[IBIS Ver]  4.0
[File Name]  lpc2478fbd.ibs
[File Rev]  1.0
[Date]  Mon Dec 18 10:34:29 2006
[Source]  Package model from Ansoft Q3D Extractor 7.1.1
[Notes]   IO models Rev 0.20 IBIS Model Design Automation Generation
[Copyright]  NXP Semiconductors 2006,2007. All rights reserved.
|   lpc2478FBD (208 LOFP package) IBIS Model
[Disclaimer]
| NXP Semiconductors warrants and represents that the IBIS models
| identified herein are owned by NXP Semiconductors (NXP).  The
| models provided are not warranted as fully representing all of the
| operating characteristics and specifications of the semiconductor
| products to which the models relate.  Moreover, unless there is a
| signed, written agreement to the contrary, these models are furnished
| on an "as is" basis without support or warranty of any kind, either
| expressed or implied, regarding the use thereof, and NXP
| specifically disclaims all implied warranties of merchantability and
| fitness of the models for any purpose.
| NXP does not assume any liability arising out of the application
| or use of these IBIS models including infringement of patents and
| copyrights, nor does NXP convey any license under its patents and
| copyrights or the rights of others.
| NXP provides IBIS models as a service to our customers.  You and
| your company shall not distribute, convey, sell, or give these models
| to anyone else without receiving prior written permission from
| NXP.
[Define Package Model]  LQFP208
[Manufacturer]  NXP Semiconductors
[OEM]  NXP
[Description]  LQFP208
|Sim freq: 100 MHz
|Date: 121806
[Number Of Pins]  208
[Pin Numbers]
1   | pin1 = lead1
2   | pin2 = lead2
3   | pin3 = lead3
4   | pin4 = lead4
5   | pin5 = lead5
6   | pin6 = lead6
7   | pin7 = lead7
8   | pin8 = lead8
9   | pin9 = lead9
10   | pin10 = lead10
11   | pin11 = lead11
12   | pin12 = lead12
13   | pin13 = lead13
14   | pin14 = lead14
15   | pin15 = lead15
16   | pin16 = lead16
17   | pin17 = lead17
18   | pin18 = lead18
19   | pin19 = lead19
20   | pin20 = lead20
21   | pin21 = lead21
22   | pin22 = lead22
23   | pin23 = lead23
24   | pin24 = lead24
25   | pin25 = lead25
26   | pin26 = lead26
27   | pin27 = lead27
28   | pin28 = lead28
29   | pin29 = lead29
30   | pin30 = lead30
31   | pin31 = lead31
32   | pin32 = lead32
33   | pin33 = lead33
34   | pin34 = lead34
35   | pin35 = lead35
36   | pin36 = lead36
37   | pin37 = lead37
38   | pin38 = lead38
39   | pin39 = lead39
40   | pin40 = lead40
41   | pin41 = lead41
42   | pin42 = lead42
43   | pin43 = lead43
44   | pin44 = lead44
45   | pin45 = lead45
46   | pin46 = lead46
47   | pin47 = lead47
48   | pin48 = lead48
49   | pin49 = lead49
50   | pin50 = lead50
51   | pin51 = lead51
52   | pin52 = lead52
53   | pin53 = lead53
54   | pin54 = lead54
55   | pin55 = lead55
56   | pin56 = lead56
57   | pin57 = lead57
58   | pin58 = lead58
59   | pin59 = lead59
60   | pin60 = lead60
61   | pin61 = lead61
62   | pin62 = lead62
63   | pin63 = lead63
64   | pin64 = lead64
65   | pin65 = lead65
66   | pin66 = lead66
67   | pin67 = lead67
68   | pin68 = lead68
69   | pin69 = lead69
70   | pin70 = lead70
71   | pin71 = lead71
72   | pin72 = lead72
73   | pin73 = lead73
74   | pin74 = lead74
75   | pin75 = lead75
76   | pin76 = lead76
77   | pin77 = lead77
78   | pin78 = lead78
79   | pin79 = lead79
80   | pin80 = lead80
81   | pin81 = lead81
82   | pin82 = lead82
83   | pin83 = lead83
84   | pin84 = lead84
85   | pin85 = lead85
86   | pin86 = lead86
87   | pin87 = lead87
88   | pin88 = lead88
89   | pin89 = lead89
90   | pin90 = lead90
91   | pin91 = lead91
92   | pin92 = lead92
93   | pin93 = lead93
94   | pin94 = lead94
95   | pin95 = lead95
96   | pin96 = lead96
97   | pin97 = lead97
98   | pin98 = lead98
99   | pin99 = lead99
100   | pin100 = lead100
101   | pin101 = lead101
102   | pin102 = lead102
103   | pin103 = lead103
104   | pin104 = lead104
105   | pin105 = lead105
106   | pin106 = lead106
107   | pin107 = lead107
108   | pin108 = lead108
109   | pin109 = lead109
110   | pin110 = lead110
111   | pin111 = lead111
112   | pin112 = lead112
113   | pin113 = lead113
114   | pin114 = lead114
115   | pin115 = lead115
116   | pin116 = lead116
117   | pin117 = lead117
118   | pin118 = lead118
119   | pin119 = lead119
120   | pin120 = lead120
121   | pin121 = lead121
122   | pin122 = lead122
123   | pin123 = lead123
124   | pin124 = lead124
125   | pin125 = lead125
126   | pin126 = lead126
127   | pin127 = lead127
128   | pin128 = lead128
129   | pin129 = lead129
130   | pin130 = lead130
131   | pin131 = lead131
132   | pin132 = lead132
133   | pin133 = lead133
134   | pin134 = lead134
135   | pin135 = lead135
136   | pin136 = lead136
137   | pin137 = lead137
138   | pin138 = lead138
139   | pin139 = lead139
140   | pin140 = lead140
141   | pin141 = lead141
142   | pin142 = lead142
143   | pin143 = lead143
144   | pin144 = lead144
145   | pin145 = lead145
146   | pin146 = lead146
147   | pin147 = lead147
148   | pin148 = lead148
149   | pin149 = lead149
150   | pin150 = lead150
151   | pin151 = lead151
152   | pin152 = lead152
153   | pin153 = lead153
154   | pin154 = lead154
155   | pin155 = lead155
156   | pin156 = lead156
157   | pin157 = lead157
158   | pin158 = lead158
159   | pin159 = lead159
160   | pin160 = lead160
161   | pin161 = lead161
162   | pin162 = lead162
163   | pin163 = lead163
164   | pin164 = lead164
165   | pin165 = lead165
166   | pin166 = lead166
167   | pin167 = lead167
168   | pin168 = lead168
169   | pin169 = lead169
170   | pin170 = lead170
171   | pin171 = lead171
172   | pin172 = lead172
173   | pin173 = lead173
174   | pin174 = lead174
175   | pin175 = lead175
176   | pin176 = lead176
177   | pin177 = lead177
178   | pin178 = lead178
179   | pin179 = lead179
180   | pin180 = lead180
181   | pin181 = lead181
182   | pin182 = lead182
183   | pin183 = lead183
184   | pin184 = lead184
185   | pin185 = lead185
186   | pin186 = lead186
187   | pin187 = lead187
188   | pin188 = lead188
189   | pin189 = lead189
190   | pin190 = lead190
191   | pin191 = lead191
192   | pin192 = lead192
193   | pin193 = lead193
194   | pin194 = lead194
195   | pin195 = lead195
196   | pin196 = lead196
197   | pin197 = lead197
198   | pin198 = lead198
199   | pin199 = lead199
200   | pin200 = lead200
201   | pin201 = lead201
202   | pin202 = lead202
203   | pin203 = lead203
204   | pin204 = lead204
205   | pin205 = lead205
206   | pin206 = lead206
207   | pin207 = lead207
208   | pin208 = lead208
[Model Data]
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[End Model Data]
[End Package Model]
|| [End]
[Component]   lpc2478FBD
[Manufacturer]  NXP
[Package]
|   typ   min   max
R_pkg   0   0   0  |Values included in package model
L_pkg   0   0   0  |Values included in package model
C_pkg   0   0   0  |Values included in package model
[Package Model]  LQFP208
| (Pin and IO model definitions)
| IMPORTANT NOTES:
| The lpc2478 GPIO pins, excluding the I2C and USB, have programmable input
| configurations. For this reason, three models are supplied for those basic
| padcells. Each model is identified by a unique suffix code at the end of
| the modelname:
| _p=plain input, _pd=pulldown enabled, _pu=pullup enabled
| The model_name for each of the GPIO pins in the [Pin] table below reflects
| the default state of that pin on power up (input with pullup enabled).
| The user may modify the model_name for a specific P#.# pin if that pin's
| input configuration is programmed differently from the default in the
| actual application. However, the model_names for all other pins are
| non-configurable and should not be altered.
| All GPIO padcells have 5ns slew rate control when operated as outputs,
| unless otherwise noted.
[Pin]   signal_name   model_name   | comments
1   P3.12   bpts5ptpht5v_pu   |
2   TDO   bpts5ptpht5v_p   | 3-state output only
3   P3.3   bpts5ptpht5v_pu   |
4   TDI   bpts5ptpht5v_pu   | In only
5   P3.28   bpts5ptpht5v_pu   |
6   TMS   bpts5ptpht5v_pu   | In only
7   P3.13   bpts5ptpht5v_pu   |
8   TRST_N   bpts5ptpht5v_pu   | In only
9   DBGEN   bpts5ptpht5v_pu   | In only
10   TCK   bpts5ptpht5v_p   | In only
11   P3.29   bpts5ptpht5v_pu   |
12   P0.26   bpats5thpept5v_pu |
13   P3.4   bpts5ptpht5v_pu   |
14   P0.25   bpats5thpept5v_pu |
15   Vdd   POWER
16   P0.24   bpats5thpept5v_pu |
17   P3.5   bpts5ptpht5v_pu   |
18   P0.23   bpats5thpept5v_pu |
19   P3.30   bpts5ptpht5v_pu   |
20   VddA   POWER
21   P3.14   bpts5ptpht5v_pu   |
22   VssA   GND
23   P3.6   bpts5ptpht5v_pu   |
24   VrefA   POWER
25   P3.31   bpts5ptpht5v_pu   |
26   Vdd   POWER   |
27   P3.7   bpts5ptpht5v_pu   |
28   P3.15   bpts5ptpht5v_pu   |
29   RSTOUTN   bpts5ptpht5v_pu   | Output only
30   Vddcore   NC   |
31   P2.30   bpts5ptpht5v_pu   |
32   Vss   GND
33   Vss   GND
34   RTCX1   NC
35   NRESET   bpts5ptpht5v_pu   | In only
36   RTCX2   NC
37   ALARM   bptpcph1v8   | Output only, 1.8V, no slew
38   VBAT   POWER
39   P2.31   bpts5ptpht5v_pu   |
40   P1.31   bpats5thpept5v_pu |
41   P0.12   bpats5thpept5v_pu |
42   P1.30   bpats5thpept5v_pu |
43   P2.29   bpts5ptpht5v_pu   |
44   X1   NC
45   P0.13   bpats5thpept5v_pu |
46   X2   NC
47   P2.27   bpts5ptpht5v_pu   |
48   P0.28   iic3m4sdat5v_400k | I2C padcell
49   P2.28   bpts5ptpht5v_pu   |
50   P0.27   iic3m4sdat5v_400k | I2C padcell
51   P0.31   usb11f1_iop_hs   | USB padcell
52   DMB   usb11f1_iom_hs   | USB padcell
53   P2.24   bpts5ptpht5v_pu   |
54   P2.25   bpts5ptpht5v_pu   |
55   P3.26   bpts5ptpht5v_pu   |
56   P3.25   bpts5ptpht5v_pu   |
57   P2.26   bpts5ptpht5v_pu   |
58   P3.24   bpts5ptpht5v_pu   |
59   P2.18   bpts5ptpht5v_pu   |
60   Vdd   POWER
61   P0.29   usb11f1_iop_hs   | USB padcell
62   P0.30   usb11f1_iom_hs   | USB padcell
63   Vss   GND
64   P2.23   bpts5ptpht5v_pu   |
65   P3.23   bpts5ptpht5v_pu   |
66   P1.18   bpts5ptpht5v_pu   |
67   P2.19   bpts5ptpht5v_pu   |
68   P1.19   bpts5ptpht5v_pu   |
69   P0.14   bpts5ptpht5v_pu   |
70   P1.20   bpts5ptpht5v_pu   |
71   Vdd   POWER
72   P1.21   bpts5ptpht5v_pu   |
73   P2.20   bpts5ptpht5v_pu   |
74   P1.22   bpts5ptpht5v_pu   |
75   P4.0   bpts5ptpht5v_pu   |
76   P1.23   bpts5ptpht5v_pu   |
77   Vss   GND
78   P1.24   bpts5ptpht5v_pu   |
79   P4.1   bpts5ptpht5v_pu   |
80   P1.25   bpts5ptpht5v_pu   |
81   P2.21   bpts5ptpht5v_pu   |
82   P1.26   bpts5ptpht5v_pu   |
83   P4.2   bpts5ptpht5v_pu   |
84   Vss   GND
85   P2.22   bpts5ptpht5v_pu   |
86   Vdd   POWER
87   P2.16   bpts5ptpht5v_pu   |
88   P1.27   bpts5ptpht5v_pu   |
89   Vdd   POWER
90   P1.28   bpts5ptpht5v_pu   |
91   P2.14   bpts5ptpht5v_pu   |
92   P1.29   bpts5ptpht5v_pu   |
93   Vss   GND
94   P0.0   bpts5ptpht5v_pu   |
95   P2.17   bpts5ptpht5v_pu   |
96   P0.1   bpts5ptpht5v_pu   |
97   P4.3   bpts5ptpht5v_pu   |
98   P0.10   bpts5ptpht5v_pu   |
99   P2.15   bpts5ptpht5v_pu   |
100   P0.11   bpts5ptpht5v_pu   |
101   P4.16   bpts5ptpht5v_pu   |
102   P2.13   bpts5ptpht5v_pu   |
103   P4.4   bpts5ptpht5v_pu   |
104   P4.17   bpts5ptpht5v_pu   |
105   P4.18   bpts5ptpht5v_pu   |
106   P2.12   bpts5ptpht5v_pu   |
107   P4.5   bpts5ptpht5v_pu   |
108   P2.11   bpts5ptpht5v_pu   |
109   P4.20   bpts5ptpht5v_pu   |
110   P2.10   bpts5ptpht5v_pu   |
111   P4.19   bpts5ptpht5v_pu   |
112   Vdd   POWER
113   P4.6   bpts5ptpht5v_pu   |
114   Vss   GND
115   P4.21   bpts5ptpht5v_pu   |
116   P0.22   bpts5ptpht5v_pu   |
117   Vddcore   NC
118   P0.21   bpts5ptpht5v_pu   |
119   P4.26   bpts5ptpht5v_pu   |
120   P0.20   bpts5ptpht5v_pu
121   P4.7   bpts5ptpht5v_pu   |
122   P0.19   bpts5ptpht5v_pu   |
123   P4.22   bpts5ptpht5v_pu   |
124   P0.18   bpts5ptpht5v_pu   |
125   Vdd   POWER
126   P0.17   bpts5ptpht5v_pu   |
127   P4.8   bpts5ptpht5v_pu   |
128   P0.15   bpts5ptpht5v_pu   |
129   P4.23   bpts5ptpht5v_pu   |
130   P0.16   bpts5ptpht5v_pu   |
131   P4.9   bpts5ptpht5v_pu   |
132   P2.9   bpts5ptpht5v_pu   |
133   Vss   GND
134   P2.8   bpts5ptpht5v_pu   |
135   P4.10   bpts5ptpht5v_pu   |
136   P2.7   bpts5ptpht5v_pu   |
137   P3.16   bpts5ptpht5v_pu   |
138   P2.6   bpts5ptpht5v_pu   |
139   P4.27   bpts5ptpht5v_pu   |
140   P2.5   bpts5ptpht5v_pu   |
141   Vddcore   NC
142   P2.4   bpts5ptpht5v_pu   |
143   P3.17   bpts5ptpht5v_pu   |
144   P2.3   bpts5ptpht5v_pu   |
145   P4.11   bpts5ptpht5v_pu   |
146   Vdd   POWER
147   P1.13   bpts5ptpht5v_pu   |
148   Vss   GND
149   P4.12   bpts5ptpht5v_pu   |
150   P2.2   bpts5ptpht5v_pu   |
151   P3.18   bpts5ptpht5v_pu   |
152   P2.1   bpts5ptpht5v_pu   |
153   P1.7   bpts5ptpht5v_pu   |
154   P2.0   bpts5ptpht5v_pu   |
155   P4.13   bpts5ptpht5v_pu   |
156   P1.5   bpts5ptpht5v_pu   |
157   P1.12   bpts5ptpht5v_pu   |
158   P0.9   bpts5ptpht5v_pu   |
159   P4.14   bpts5ptpht5v_pu   |
160   P0.8   bpts5ptpht5v_pu   |
161   P3.19   bpts5ptpht5v_pu   |
162   P0.7   bpts5ptpht5v_pu   |
163   P1.11   bpts5ptpht5v_pu   |
164   P0.6   bpts5ptpht5v_pu   |
165   Vdd   POWER
166   P0.5   bpts5ptpht5v_pu   |
167   P3.20   bpts5ptpht5v_pu   |
168   P0.4   bpts5ptpht5v_pu   |
169   Vss   GND
170   P4.28   bpts5ptpht5v_pu   |
171   P1.6   bpts5ptpht5v_pu   |
172   Vss   GND
173   P4.15   bpts5ptpht5v_pu   |
174   Vdd   POWER
175   P3.21   bpts5ptpht5v_pu   |
176   P4.29   bpts5ptpht5v_pu   |
177   P1.3   bpts5ptpht5v_pu   |
178   P1.17   bpts5ptpht5v_pu   |
179   P4.25   bpts5ptpht5v_pu   |
180   P1.16   bpts5ptpht5v_pu   |
181   Vdd   POWER
182   P1.15   bpts5ptpht5v_pu   |
183   P4.24   bpts5ptpht5v_pu   |
184   P1.14   bpts5ptpht5v_pu   |
185   P1.2   bpts5ptpht5v_pu   |
186   P1.10   bpts5ptpht5v_pu   |
187   P4.30   bpts5ptpht5v_pu   |
188   P1.9   bpts5ptpht5v_pu   |
189   Vss   GND
190   P1.8   bpts5ptpht5v_pu   |
191   P3.8   bpts5ptpht5v_pu   |
192   P1.4   bpts5ptpht5v_pu   |
193   P4.31   bpts5ptpht5v_pu   |
194   P1.1   bpts5ptpht5v_pu   |
195   P3.22   bpts5ptpht5v_pu   |
196   P1.0   bpts5ptpht5v_pu   |
197   P3.0   bpts5ptpht5v_pu   |
198   Vdd   POWER
199   P3.9   bpts5ptpht5v_pu   |
200   Vss   GND
201   P3.1   bpts5ptpht5v_pu   |
202   P0.2   bpts5ptpht5v_pu   |
203   P3.27   bpts5ptpht5v_pu   |
204   P0.3   bpts5ptpht5v_pu   |
205   P3.10   bpts5ptpht5v_pu   |
206   RTCK   bpts5ptpht5v_pu   |
207   P3.2   bpts5ptpht5v_pu   |
208   P3.11   bpts5ptpht5v_pu   |
| Models and submodels in the file (10): bpats5thpept5v_p (I/O), bpats5thpept5v_pd (I/O), bpats5thpept5v_pu (I/O), bpts5ptpht5v_p (I/O), bpts5ptpht5v_pd (I/O), bpts5ptpht5v_pu (I/O), iic3m4sdat5v_400k (I/O_open_drain), usb11f1_iom_hs (I/O), usb11f1_iop_hs (I/O), bptpcph1v8 (Output)
